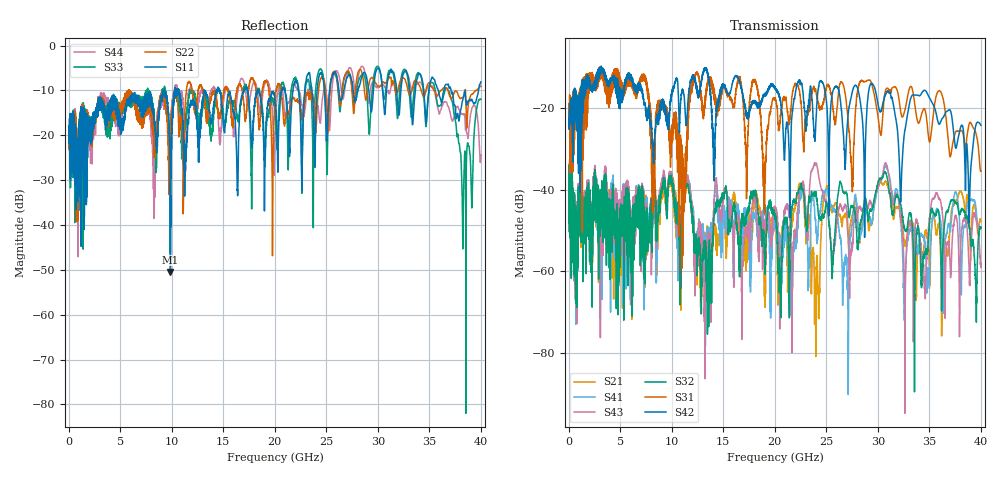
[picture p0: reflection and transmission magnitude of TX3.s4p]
!Agilent Technologies,N5245A,MY49151084,A.09.00.04
!Agilent N5245A: A.09.00.04
!Date: Thursday, January 20, 2011 08:30:43
!Correction: S11(Full 4 Port(1,2,3,4))
!S12(Full 4 Port(1,2,3,4))
!S13(Full 4 Port(1,2,3,4))
!S14(Full 4 Port(1,2,3,4))
!S21(Full 4 Port(1,2,3,4))
!S22(Full 4 Port(1,2,3,4))
!S23(Full 4 Port(1,2,3,4))
!S24(Full 4 Port(1,2,3,4))
!S31(Full 4 Port(1,2,3,4))
!S32(Full 4 Port(1,2,3,4))
!S33(Full 4 Port(1,2,3,4))
!S34(Full 4 Port(1,2,3,4))
!S41(Full 4 Port(1,2,3,4))
!S42(Full 4 Port(1,2,3,4))
!S43(Full 4 Port(1,2,3,4))
!S44(Full 4 Port(1,2,3,4))
!S4P File: Measurements: <S11,S12,S13,S14>,
!<S21,S22,S23,S24>,
!<S31,S32,S33,S34>,
!<S41,S42,S43,S44>:
# Hz S  dB  R 50
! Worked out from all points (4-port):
!   3996 points, 50 MHz to 40 GHz, reference 50 ohm
!   strongest paths, dB at 50 MHz, 10.04 GHz, 20.03 GHz, 30.02 GHz, 40 GHz:
!     S42: -22.4, -15.6, -15.1, -19.0, -24.2
!     S31: -21.8, -24.7, -17.5, -22.0, -35.4
!     S32: -50.3, -37.7, -45.9, -38.3, -49.3
!     S43: -49.4, -37.5, -45.3, -39.7, -59.1
!     S41: -49.8, -38.6, -48.2, -39.3, -49.2
!     S21: -50.0, -38.4, -48.1, -38.3, -47.7
!   lowest |S11| = -50.5 dB at 9.88 GHz (marker M1), VSWR 1.01, Z = 50 + j0.299 ohm
!   |S11| at or under -10 dB: start of sweep to 9.276 GHz; 10.74 GHz to 13.17 GHz (2.434 GHz wide, 20.4 % of centre); 37.1 GHz to 39.77 GHz (2.668 GHz wide, 6.94 % of centre)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
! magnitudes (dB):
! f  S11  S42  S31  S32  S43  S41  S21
! 50 MHz  -18.8  -22.4  -21.8  -50.3  -49.4  -49.8  -50.0
! 9.88 GHz  -50.5  -18.0  -30.4  -38.3  -37.5  -37.4  -38.1
! 13.26 GHz  -10.2  -10.1  -16.9  -53.6  -57.9  -57.1  -55.6
! 22.49 GHz  -14.8  -13.9  -17.7  -39.8  -39.1  -41.4  -38.9
! 24.13 GHz  -9.7  -17.3  -17.5  -43.6  -34.5  -51.5  -59.5
! 25.06 GHz  -21.2  -19.6  -14.7  -43.5  -43.3  -39.8  -39.1
! 40 GHz  -8.1  -24.2  -35.4  -49.3  -59.1  -49.2  -47.7
